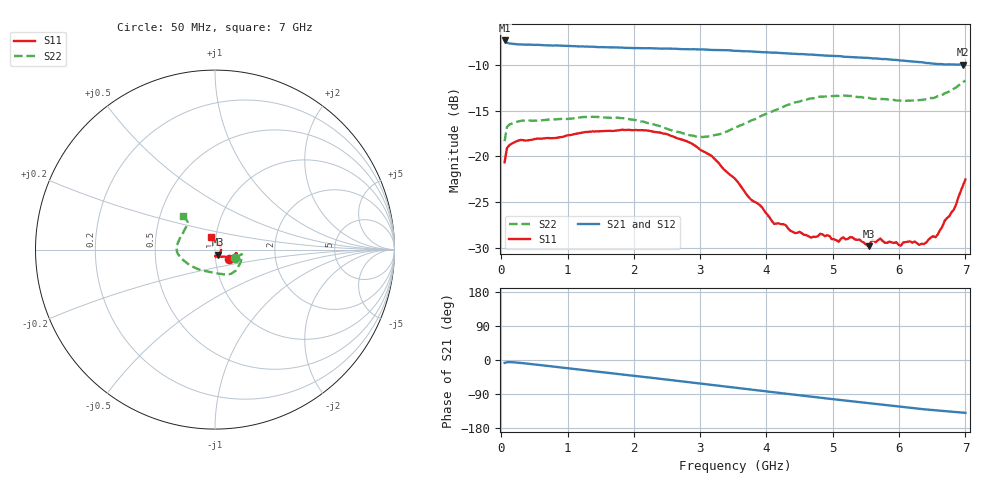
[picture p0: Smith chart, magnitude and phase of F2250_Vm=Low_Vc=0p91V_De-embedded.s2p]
! Integrated Device Technology
! Corporate Headquarters
! 6024 Silver Creek Valley Road
! San Jose, CA 95138  USA
! Phone:  1-408-284-8200
! Toll Free:  1-800-223-1366
! Webpage:  http://www.idt.com/
! Timing and RF Division
! 515 Groton Road, Suite 102
! Westford, MA 01886-6024
! Device:  F2250
! Description: Voltage Variable RF Attenuator
! Frequency:  50.0 -  6000.00 MHz
! Package:  3x3 mm Thin QFN Plastic Package: 16 pin
! Ports:  2 RF, 3 DC
!  Pin  1  = GND
!  Pin  2  = NC
!  Pin  3  = RF1  = Port 1
!  Pin  4  = NC
!  Pin  5  = GND
!  Pin  6  = GND
!  Pin  7  = GND
!  Pin  8  = GND
!  Pin  9  = NC
!  Pin 10  = RF2  = Port 2
!  Pin 11  = NC
!  Pin 12  = GND
!  Pin 13  = GND
!  Pin 14  = VCNTRL
!  Pin 15  = VDD
!  Pin 16  = VMODE
! Vcntrl:  0.910 Volts
! Vmode:  +0.000 Volts
! Vdd:  +3.30  Volts
! Current:  1.178 mA
! Data:  The device was measured on a the F2250 evaluation board which has
!  individual transmission lines to the RF pins.  Data was collected
!  using a calibrated network analyzer.  The evaluation board was
!  de-embedded using a TRL calibration technique.
!  The reference plane is the edge of the package pin.
! Misc:  SN 10
!  Action Tracker AT0258
! Date Measured:  2014-11-26
! Date:  2015-10-15  MJV
! Note:
!  Integrated Device Technology supplies this data as a sample of measured
!  data at the package pin for this product.  Your particular data for this
!  product may vary.
!  Data was taken at 25 degrees C.
!  Integrated Device Technology reserves the right to change this data at anytime.
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# GHz S dB R 50
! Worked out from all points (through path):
!   201 points, 50 MHz to 7 GHz, reference 50 ohm
!   highest |S21| = -7.32 dB at 50 MHz (marker M1); lowest = -10.0 dB at 6.965 GHz (marker M2)
!   group delay of S21, straight-line fit = 55.8 ps
!   lowest |S11| = -29.8 dB at 5.54 GHz (marker M3), VSWR 1.07, Z = 51.5 - j2.88 ohm
!   |S11| at or under -10 dB: start of sweep to end of sweep
!   |S22| runs from -18.3 to -11.7 dB; largest |S21 - S12| = 0.0011
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0.05  -20.65 -32.4  -7.32 -7.6  -7.31 -7.6  -18.34 -21.9
0.08475  -19.12 -16.2  -7.56 -5.9  -7.56 -5.9  -16.81 -12.1
0.2585  -18.27 -9.5  -7.74 -7.2  -7.74 -7.2  -16.20 -12.7
1.2315  -17.39 -23.0  -7.96 -26.4  -7.96 -26.4  -15.70 -42.2
1.857  -17.12 -25.1  -8.12 -38.8  -8.11 -38.8  -15.84 -56.7
2.37825  -17.38 -24.5  -8.20 -49.3  -8.19 -49.3  -16.67 -70.2
2.79525  -18.34 -24.6  -8.27 -57.8  -8.27 -57.8  -17.59 -87.6
3.0385  -19.44 -26.1  -8.29 -62.9  -8.29 -62.9  -17.89 -101.6
3.525  -22.46 -34.2  -8.45 -73.0  -8.44 -73.1  -16.87 -130.6
4.11575  -27.40 -60.9  -8.65 -85.3  -8.65 -85.3  -15.00 -157.2
4.7065  -28.81 -86.8  -8.88 -97.4  -8.88 -97.4  -13.65 -173.6
4.81075  -28.49 -87.4  -8.93 -99.4  -8.93 -99.5  -13.48 -175.6
5.08875  -29.36 -83.6  -9.03 -105.1  -9.03 -105.1  -13.39 177.8
5.2625  -28.84 -75.3  -9.13 -108.5  -9.12 -108.5  -13.39 173.9
5.5405  -29.85 -60.1  -9.24 -114.0  -9.23 -114.0  -13.60 166.9
5.61  -29.18 -54.5  -9.28 -115.4  -9.26 -115.4  -13.72 165.2
5.85325  -29.35 -36.8  -9.40 -120.1  -9.40 -120.2  -13.81 158.8
6.305  -29.70 13.4  -9.69 -128.7  -9.68 -128.7  -13.85 144.1
6.54825  -28.87 48.8  -9.87 -132.7  -9.87 -132.7  -13.54 137.1
6.82625  -25.83 87.6  -9.95 -136.8  -9.94 -136.8  -12.60 133.8
6.96525  -23.19 105.2  -9.97 -139.0  -9.96 -139.0  -11.89 133.8
7  -22.55 108.0  -9.95 -139.5  -9.94 -139.6  -11.68 133.4
